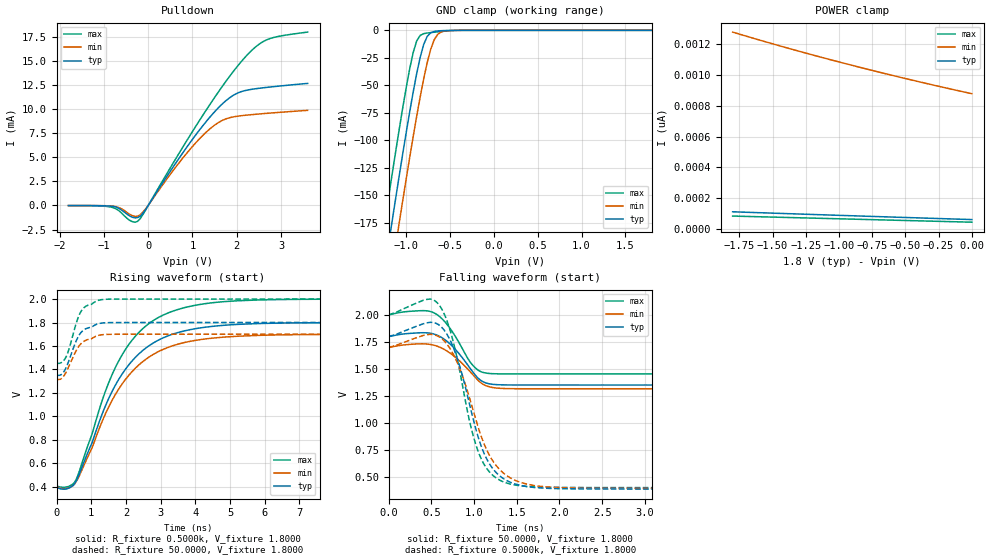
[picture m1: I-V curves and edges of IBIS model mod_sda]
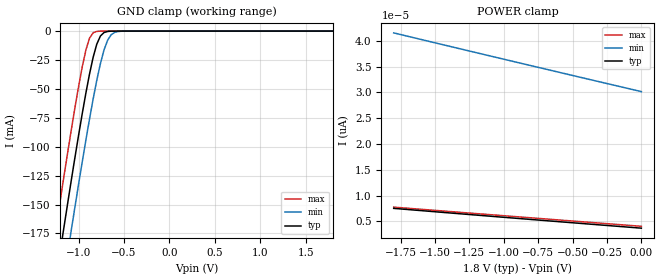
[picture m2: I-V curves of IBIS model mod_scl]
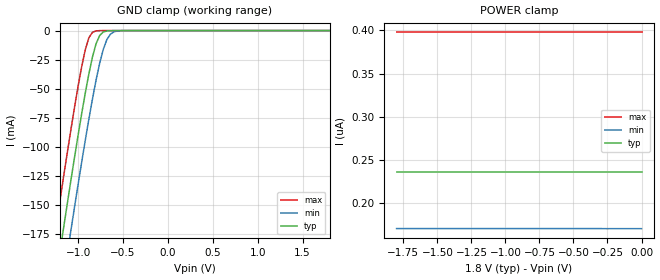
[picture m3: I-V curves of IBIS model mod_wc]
| IBIS (I/O, Buffer, Information, Specification) Model, officially
| electronic behavioral standard for Buffer structures of digital pins.
[IBIS ver]  4.0
[File name] m24c08_fb1_tssop8.ibs
[File Rev]  1.0
[Date]   23 May 2014
[Source]   CAD & Design Services (Catania) - STMicroelectronics
[Notes]
   (Note1)  This IBIS model includes the SO8 package data
   (Note2)  This IBIS model has some Notes about the non-monotonicity
   of the I-V curves, but they are not indicative of problems
   inside the model;
[Copyright] (c) 2014 STMicroelectronics
|   Component M24C16
[Component] M24C16
[Manufacturer] STMicroelectronics
[Package]
| variable   typ   min   max
R_pkg   0.0   0.0   0.0
L_pkg   0.0H   0.0H   0.0H
C_pkg   0.0F   0.0F   0.0F
[Pin]  signal_name   model_name   R_pin   L_pin   C_pin
1   1NC   NC   NA   NA   NA
2   2NC   NC   NA   NA   NA
3   3NC   NC   NA   NA   NA
4   VSS   GND   NA   NA   NA
5   SDA   mod_sda   NA   NA   NA
6   SCL   mod_scl   NA   NA   NA
7   WCN   mod_wc   NA   NA   NA
8   VCC   POWER   NA   NA   NA
[Package Model]  182696_TSSOP8
[Define Package Model]  182696_TSSOP8
[Manufacturer]  STMicroelectronics
[OEM]  STMicroelectronics
[Description]  8 pin TSSOP package
[Number Of Pins]  8
[Pin Numbers]
|Pin Num   Terminal Name
1   | net1
2   | net2
3   | net3
4   | net4_GND
5   | net5
6   | net6
7   | net7
8   | net8_VDD
[Model Data]
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[End Model Data]
[End Package Model]
| Models and submodels in the file (3): mod_sda (I/O_open_drain), mod_scl (Input), mod_wc (Input)
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|   Model mod_sda
[Model]   mod_sda
Model_type I/O_open_drain
Polarity   Non-Inverting
Vinl   =   0.540V
Vinh   =   1.260V
Vmeas  =   0.900V
Cref   =   10pF
Rref   =   1k
Vref   =   1.800V
C_comp   2.024pF   1.845pF   2.119pF
[Temperature Range]  25.0000   85.0000   -40.0000
[Voltage Range]   1.8000V   1.7000V   2.0000V
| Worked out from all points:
|   slope of the pulldown table from 0 to 0.27 V, typ, clamps not added: 138 ohm
|   GND clamp passes 1 mA (typ) near -0.68 V on its own axis
|   rising waveform, R_fixture 0.5000k, V_fixture 1.8000: 20-80 % time 1.45ns typ, 1.47ns min, 1.39ns max; typ from 0.392 V to 1.8 V
|   rising waveform, R_fixture 50.0000, V_fixture 1.8000: 20-80 % time 380ps typ, 414ps min, 349ps max; typ from 1.35 V to 1.8 V
|   falling waveform, R_fixture 50.0000, V_fixture 1.8000: 20-80 % time 272ps typ, 291ps min, 252ps max; typ from 1.8 V to 1.35 V
|   falling waveform, R_fixture 0.5000k, V_fixture 1.8000: 20-80 % time 312ps typ, 352ps min, 277ps max; typ from 1.8 V to 0.392 V
[Pulldown]
|Voltage   I(typ)   I(min)   I(max)
-1.8V     -5.1uA     -3.444uA   -16.54uA
-840mV    -67.22uA   -45.2uA    -164.2uA
-420mV    -1.078mA   -910.8uA   -1.532mA
-240mV    -1.259mA   -1.115mA   -1.653mA
-60mV     -440.2uA   -355.5uA   -477.5uA
1.08V     7.363mA    6.534mA    8.26mA
1.5V      9.727mA    8.339mA    11.21mA
1.8V      11.04mA    9.057mA    13.17mA
2.22V     11.96mA    9.377mA    15.55mA
2.58V     12.21mA    9.526mA    16.97mA
2.88V     12.36mA    9.635mA    17.49mA
3.6V      12.67mA    9.873mA    17.99mA
[GND_clamp]
|Voltage   I(typ)   I(min)   I(max)
-1.8V     -517.5mA   -559.9mA   -476mA
-1.28V    -236.5mA   -279.7mA   -193.8mA
-1.24V    -215.4mA   -258.6mA   -172.7mA
-1.16V    -173.7mA   -216.8mA   -131mA
-1.08V    -132.8mA   -175.7mA   -90.53mA
-920mV    -56.25mA   -96.78mA   -20.32mA
-840mV    -24.6mA    -60.61mA   -4.609mA
-800mV    -12.91mA   -44.14mA   -3.035mA
-720mV    -2.232mA   -17.25mA   -2.057mA
-680mV    -1.036mA   -8.577mA   -1.696mA
-600mV    -344.1uA   -1.488mA   -1.014mA
1.8V      61.17pA    897pA      39.74pA
[POWER_clamp]
|Voltage   I(typ)   I(min)   I(max)
-1.8V     111.7pA    1.278nA    83.87pA
-1.38V    99.45pA    1.173nA    74.58pA
-920mV    86.39pA    1.066nA    64.42pA
-460mV    73.64pA    968.3pA    54.28pA
0V        61.17pA    878pA      44.14pA
[Ramp]
| variable   typ   min   max
dV/dt_r   0.2685/0.5071n   0.2293/0.5442n   0.3271/0.4322n
dV/dt_f   0.2685/0.3169n   0.2293/0.3382n   0.3271/0.3096n
R_load = 50.0000
[Rising Waveform]
R_fixture= 0.5000k
V_fixture= 1.8000
V_fixture_min= 1.7000
V_fixture_max= 2.0000
|time   V(typ)   V(min)   V(max)
0s        392.3mV    398.1mV    405.8mV
270ps     380.1mV    382.8mV    395.8mV
520ps     424.9mV    422.5mV    437.4mV
1.01ns    764.7mV    722.2mV    837mV
1.39ns    1.075V     1.008V     1.198V
1.75ns    1.294V     1.213V     1.448V
2.29ns    1.508V     1.416V     1.689V
2.99ns    1.658V     1.56V      1.851V
4.85ns    1.777V     1.676V     1.979V
10ns      1.8V       1.7V       2V
[Rising Waveform]
R_fixture= 50.0000
V_fixture= 1.8000
V_fixture_min= 1.7000
V_fixture_max= 2.0000
|time   V(typ)   V(min)   V(max)
0s        1.353V     1.318V     1.455V
150ps     1.359V     1.324V     1.461V
270ps     1.412V     1.373V     1.504V
370ps     1.486V     1.435V     1.584V
590ps     1.658V     1.572V     1.814V
650ps     1.692V     1.6V       1.862V
730ps     1.723V     1.626V     1.906V
850ps     1.748V     1.649V     1.939V
1.27ns    1.794V     1.694V     1.994V
10ns      1.8V       1.7V       2V
[Falling Waveform]
R_fixture= 50.0000
V_fixture= 1.8000
V_fixture_min= 1.7000
V_fixture_max= 2.0000
|time   V(typ)   V(min)   V(max)
0s        1.8V       1.7V       2V
380ps     1.834V     1.732V     2.038V
540ps     1.82V      1.718V     2.014V
620ps     1.791V     1.694V     1.967V
720ps     1.73V      1.646V     1.874V
980ps     1.479V     1.454V     1.539V
1.08ns    1.395V     1.373V     1.476V
1.2ns     1.361V     1.332V     1.458V
1.6ns     1.353V     1.318V     1.455V
10ns      1.353V     1.318V     1.455V
[Falling Waveform]
R_fixture= 0.5000k
V_fixture= 1.8000
V_fixture_min= 1.7000
V_fixture_max= 2.0000
|time   V(typ)   V(min)   V(max)
0s        1.8V       1.7V       2V
430ps     1.923V     1.814V     2.14V
600ps     1.9V       1.793V     2.081V
800ps     1.607V     1.566V     1.607V
960ps     1.134V     1.2V       977.8mV
1.06ns    844.3mV    935.7mV    716.2mV
1.22ns    581.6mV    653.2mV    519.7mV
1.46ns    445.4mV    481.8mV    433.5mV
2.26ns    394.6mV    401.7mV    407.5mV
10ns      392.3mV    398.2mV    405.8mV
|   Model mod_scl
[Model]   mod_scl
Model_type Input
Vinl   =   0.540V
Vinh   =   1.260V
C_comp   1.763pF   1.683pF   1.933pF
[Temperature Range]  25.0000   85.0000   -40.0000
[Voltage Range]   1.8000V   1.7000V   2.0000V
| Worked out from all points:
|   GND clamp passes 1 mA (typ) near -0.71 V on its own axis
[GND_clamp]
|Voltage   I(typ)   I(min)   I(max)
-1.8V     -506.7mA   -549.3mA   -463.8mA
-1.28V    -230.6mA   -274mA     -186.5mA
-1.24V    -209.8mA   -253.3mA   -165.8mA
-1.16V    -168.9mA   -212.2mA   -124.8mA
-1.08V    -128.7mA   -171.8mA   -85.14mA
-920mV    -53.64mA   -94.29mA   -16.44mA
-840mV    -22.68mA   -58.76mA   -1.468mA
-800mV    -11.31mA   -42.6mA    -261.9uA
-720mV    -1.249mA   -16.25mA   -6.98uA
-680mV    -318.6uA   -7.797mA   -1.128uA
-600mV    -18.77uA   -1.043mA   -29.45nA
1.8V      3.674pA    30.76pA    3.627pA
[POWER_clamp]
|Voltage   I(typ)   I(min)   I(max)
-1.8V     7.509pA    41.51pA    7.748pA
-940mV    5.652pA    36.04pA    5.962pA
-440mV    4.594pA    32.89pA    4.934pA
0V        3.674pA    30.14pA    4.034pA
|   Model mod_wc
[Model]   mod_wc
Model_type Input
Vinl   =   0.540V
Vinh   =   1.260V
C_comp   1.763pF   1.683pF   1.933pF
[Temperature Range]  25.0000   85.0000   -40.0000
[Voltage Range]   1.8000V   1.7000V   2.0000V
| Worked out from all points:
|   GND clamp passes 1 mA (typ) near -0.71 V on its own axis
[GND_clamp]
|Voltage   I(typ)   I(min)   I(max)
-1.8V     -506.7mA   -549.3mA   -463.8mA
-1.28V    -230.6mA   -274mA     -186.5mA
-1.24V    -209.8mA   -253.3mA   -165.8mA
-1.16V    -168.9mA   -212.2mA   -124.8mA
-1.08V    -128.7mA   -171.8mA   -85.14mA
-920mV    -53.64mA   -94.29mA   -16.44mA
-840mV    -22.68mA   -58.76mA   -1.468mA
-800mV    -11.31mA   -42.6mA    -261.9uA
-720mV    -1.249mA   -16.25mA   -6.98uA
-680mV    -318.6uA   -7.797mA   -1.128uA
-600mV    -18.77uA   -1.043mA   -29.45nA
1.8V      3.674pA    30.76pA    3.627pA
[POWER_clamp]
|Voltage   I(typ)   I(min)   I(max)
-1.8V     235.8nA    170.8nA    397.7nA
-300mV    235.8nA    170.8nA    397.7nA
-280mV    235.8nA    170.7nA    397.7nA
0V        235.8nA    170.7nA    397.7nA
